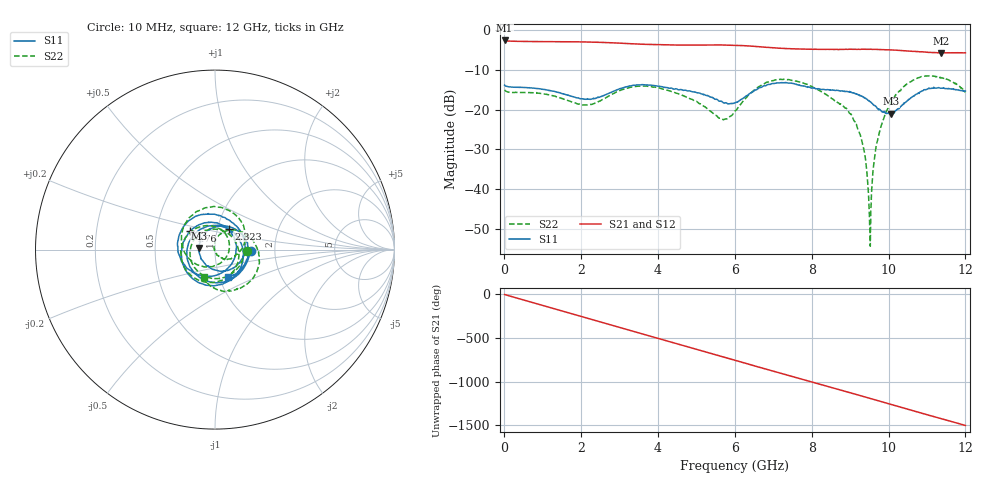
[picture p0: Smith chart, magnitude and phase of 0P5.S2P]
!Agilent Technologies,E5071C,MY46316741,A.11.02
!Date: Wed Sep 16 11:43:04 2020
!Data & Calibration Information:
!Freq	S11:SOLT2(ON)	S21:SOLT2(ON)	S12:SOLT2(ON)	S22:SOLT2(ON)
!PortZ  Port1:50+j0  Port2:50+j0
!Above PortZ is port z conversion or system Z0 setting when saving the data.
!When reading, reference impedance value at option line is always used.
# Hz S dB R 50
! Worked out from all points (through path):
!   1561 points, 10 MHz to 12 GHz, reference 50 ohm
!   highest |S21| = -2.68 dB at 10 MHz (marker M1); lowest = -5.8 dB at 11.38 GHz (marker M2)
!   group delay of S21, straight-line fit = 348 ps
!   lowest |S11| = -21.1 dB at 10.06 GHz (marker M3), VSWR 1.19, Z = 41.9 + j0.761 ohm
!   |S11| at or under -10 dB: start of sweep to end of sweep
!   |S22| runs from -54.3 to -11.5 dB; largest |S21 - S12| = 0.0051
!   S11 on the Smith chart (normalised r, x): 10 MHz: 1.51, -0.03; 2.323 GHz: 1.13, +0.27; 4.76 GHz: 0.74, +0.16; 12 GHz: 1.09, -0.35
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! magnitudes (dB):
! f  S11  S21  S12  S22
! 10 MHz  -13.9  -2.7  -2.7  -15.1
! 2.016 GHz  -17.3  -3.0  -3.0  -18.8
! 2.323 GHz  -17.1  -3.1  -3.1  -18.6
! 3.223 GHz  -14.2  -3.5  -3.5  -14.6
! 4.007 GHz  -14.1  -3.8  -3.8  -14.6
! 4.76 GHz  -15.3  -3.8  -3.8  -16.9
! 5.659 GHz  -18.0  -3.8  -3.8  -22.3
! 6.005 GHz  -18.3  -3.9  -3.9  -20.4
! 6.904 GHz  -13.7  -4.5  -4.5  -12.9
! 8.011 GHz  -14.6  -4.9  -4.9  -14.3
! 8.81 GHz  -15.4  -4.9  -4.9  -19.0
! 9.118 GHz  -15.9  -4.9  -4.9  -23.0
! 9.364 GHz  -17.0  -4.9  -4.9  -30.3
! 9.425 GHz  -17.3  -4.9  -4.9  -34.6
! 9.487 GHz  -17.8  -4.9  -4.9  -43.0
! 9.517 GHz  -18.0  -4.9  -4.9  -49.2
! 9.687 GHz  -19.4  -4.9  -4.9  -28.9
! 10 GHz  -21.0  -5.0  -5.1  -19.3
! 10.06 GHz  -21.1  -5.0  -5.1  -18.3
! 10.69 GHz  -16.3  -5.4  -5.5  -12.4
! 11.38 GHz  -14.6  -5.8  -5.8  -12.1
! 12 GHz  -15.4  -5.8  -5.8  -15.7
